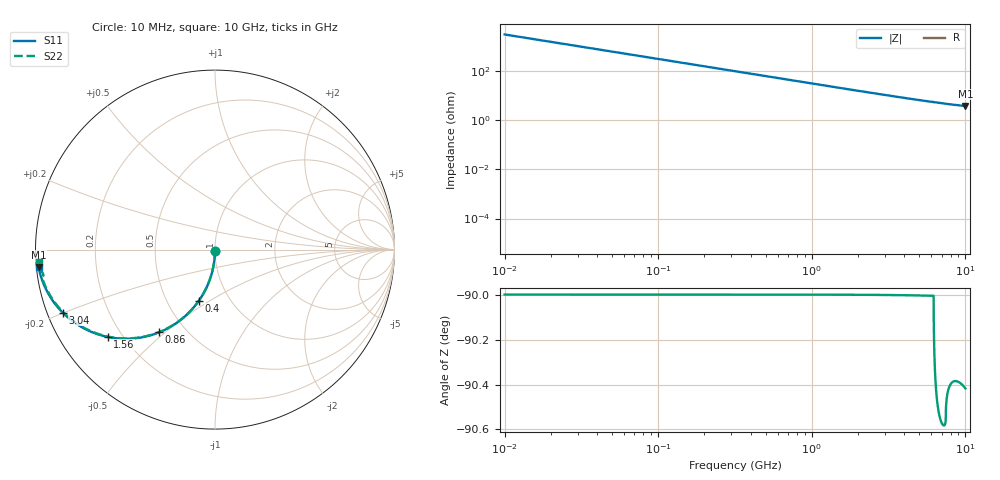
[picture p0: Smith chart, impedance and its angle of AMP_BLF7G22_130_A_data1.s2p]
! Created Thu Jul 08 13:31:27 2010
# ghz S ma R 50
! 2 Port Network Data from SP1.SP block
! freq  magS11  angS11  magS21  angS21  magS12  angS12  magS22  angS22
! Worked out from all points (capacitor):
!   1000 points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, 10 MHz to 10 GHz, reference 50 ohm
!   read as one part in shunt: C = 4.99 pF near 60 MHz
!   lowest |Z| = 3.86 ohm at 10 GHz (marker M1)
!   S11 on the Smith chart (normalised r, x): 10 MHz: 1.00, -0.02; 400 MHz: 0.72, -0.45; 860 MHz: 0.36, -0.48; 1.56 GHz: 0.15, -0.35; 3.04 GHz: 0.04, -0.20; 10 GHz: 0.01, -0.05
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0.01  0.007806 -90.4  1 -0.5  1 -0.5  0.007806 -90.4
0.03  0.02341 -91.3  0.9997 -1.4  0.9997 -1.4  0.02341 -91.4
0.07  0.05456 -93.1  0.9985 -3.2  0.9985 -3.2  0.05456 -93.2
0.08  0.06233 -93.6  0.9981 -3.6  0.9981 -3.6  0.06233 -93.6
0.1  0.07783 -94.5  0.997 -4.5  0.997 -4.5  0.07783 -94.5
0.13  0.101 -95.8  0.9949 -5.8  0.9949 -5.8  0.101 -95.9
0.18  0.1391 -98.0  0.9903 -8.1  0.9903 -8.1  0.1391 -98.1
0.24  0.1841 -100.7  0.9829 -10.7  0.9829 -10.7  0.1841 -100.7
0.31  0.2351 -103.7  0.972 -13.7  0.972 -13.7  0.2351 -103.7
0.4  0.2979 -107.4  0.9546 -17.5  0.9546 -17.5  0.2979 -107.5
0.6  0.4237 -115.2  0.9058 -25.3  0.9058 -25.3  0.4237 -115.3
0.86  0.5564 -124.0  0.8309 -34.1  0.8309 -34.1  0.5564 -124.2
1.17  0.6728 -132.6  0.7398 -42.7  0.7398 -42.7  0.6728 -132.8
1.56  0.7706 -140.8  0.6373 -51.0  0.6373 -51.0  0.7706 -141.1
1.68  0.7928 -142.9  0.6095 -53.1  0.6095 -53.1  0.7928 -143.2
2.28  0.8689 -151.0  0.495 -61.2  0.495 -61.2  0.8689 -151.4
3.04  0.9183 -157.5  0.3959 -67.8  0.3959 -67.8  0.9183 -158.1
3.34  0.9304 -159.4  0.3666 -69.7  0.3666 -69.7  0.9304 -160.1
5.01  0.9653 -166.3  0.2609 -76.8  0.2609 -76.8  0.9653 -167.4
6.67  0.9782 -170.1  0.2054 -81.4  0.2054 -81.4  0.9663 -171.6
8.34  0.9848 -172.5  0.1723 -83.6  0.1723 -83.6  0.9776 -173.9
10  0.988 -174.3  0.1525 -85.6  0.1525 -85.6  0.9815 -176.0
